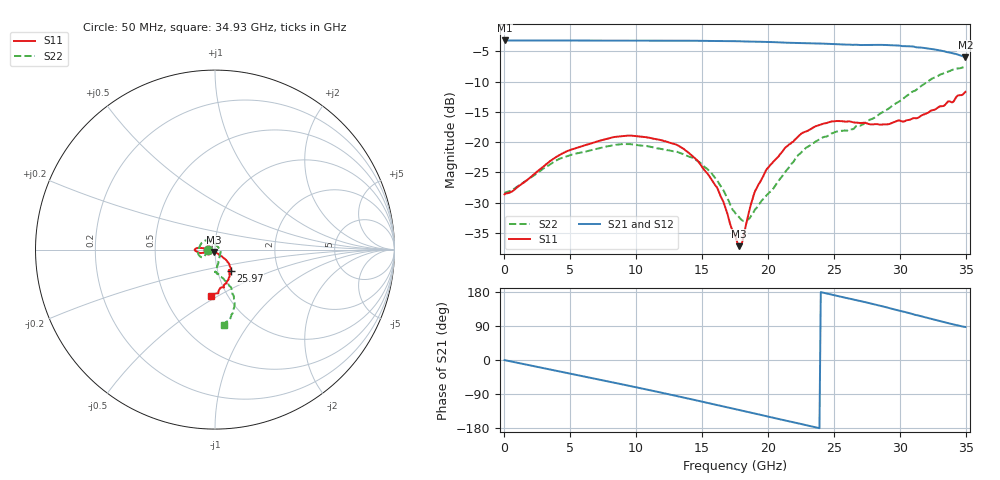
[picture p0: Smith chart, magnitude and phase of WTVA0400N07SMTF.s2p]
! 50 ohm 2-Port S-parameters measured by Modelithics Inc support@modelithics.com  Tampa, FL USA 813-866-6335 (February 2024)
! Smiths Interconnect,  4dB P/N: WTVA0400N07SMTF, Temperature: 75 C
! Board: 10 mil Rogers 4350B, Mounting Pad Dimensions: Length: 15 mils, Width: 25 mils, Gap: 40 mils.
# Hz S RI R 50
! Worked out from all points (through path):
!   352 points, 50 MHz to 34.93 GHz, reference 50 ohm
!   highest |S21| = -3.20 dB at 50 MHz (marker M1); lowest = -6.0 dB at 34.93 GHz (marker M2)
!   group delay of S21, straight-line fit = 21.7 ps
!   lowest |S11| = -37.2 dB at 17.81 GHz (marker M3), VSWR 1.03, Z = 49.5 - j1.27 ohm
!   |S11| at or under -10 dB: start of sweep to end of sweep
!   |S22| runs from -33.0 to -7.5 dB; largest |S21 - S12| = 0.008
!   S11 on the Smith chart (normalised r, x): 50 MHz: 0.93, +0.00; 25.97 GHz: 1.15, -0.28; 34.93 GHz: 0.84, -0.47
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5e7  -0.037 0.000134  0.6914 -0.00401  0.6906 -0.00382  -0.0373 -0.00157
4.18e9  -0.0755 -0.0195  0.5994 -0.3431  0.5985 -0.3428  -0.0621 -0.0381
5.8715e9  -0.0909 -0.0166  0.5133 -0.4614  0.5128 -0.4609  -0.0702 -0.0425
9.155e9  -0.1128 -0.00263  0.2823 -0.6284  0.2818 -0.6276  -0.0937 -0.0229
1.1742e10  -0.1046 0.00658  0.061 -0.6855  0.0596 -0.6848  -0.0877 0.0127
1.3135e10  -0.094 0.00921  -0.0648 -0.6849  -0.0665 -0.684  -0.0741 0.0375
1.4727e10  -0.0684 0.00841  -0.2103 -0.6541  -0.2105 -0.6532  -0.046 0.0512
1.612e10  -0.0424 0.000672  -0.3283 -0.6005  -0.3288 -0.5994  -0.021 0.0436
1.7513e10  -0.0127 -0.0108  -0.4343 -0.5258  -0.4342 -0.5248  0.00363 0.0256
1.78115e10  -0.00519 -0.0128  -0.4564 -0.5053  -0.4554 -0.505  0.00951 0.022
1.80105e10  -2.1e-05 -0.0146  -0.469 -0.4913  -0.468 -0.491  0.013 0.0186
1.8508e10  0.014 -0.0214  -0.4989 -0.4577  -0.4989 -0.4567  0.0209 0.00963
1.90055e10  0.0247 -0.0308  -0.5272 -0.4218  -0.5268 -0.4211  0.0278 0.000486
1.9901e10  0.0426 -0.0424  -0.5733 -0.3508  -0.5725 -0.3506  0.03 -0.0211
2.1294e10  0.0658 -0.0618  -0.6217 -0.2305  -0.6211 -0.2301  0.022 -0.0525
2.21895e10  0.077 -0.0772  -0.642 -0.1532  -0.6416 -0.1512  0.019 -0.0741
2.33835e10  0.0868 -0.0991  -0.653 -0.046  -0.6523 -0.0462  0.0104 -0.0972
2.59705e10  0.0871 -0.1193  -0.6129 0.1823  -0.6119 0.1824  0.00327 -0.1243
2.91545e10  0.08 -0.1162  -0.4647 0.4299  -0.46 0.4336  0.0653 -0.179
3.204e10  0.0784 -0.1553  -0.2153 0.5544  -0.2128 0.5546  0.1097 -0.2951
3.37315e10  0.0488 -0.2116  -0.0599 0.546  -0.0556 0.5457  0.0878 -0.3761
3.49255e10  -0.0201 -0.2595  0.0249 0.5015  0.0251 0.5006  0.0528 -0.4179
